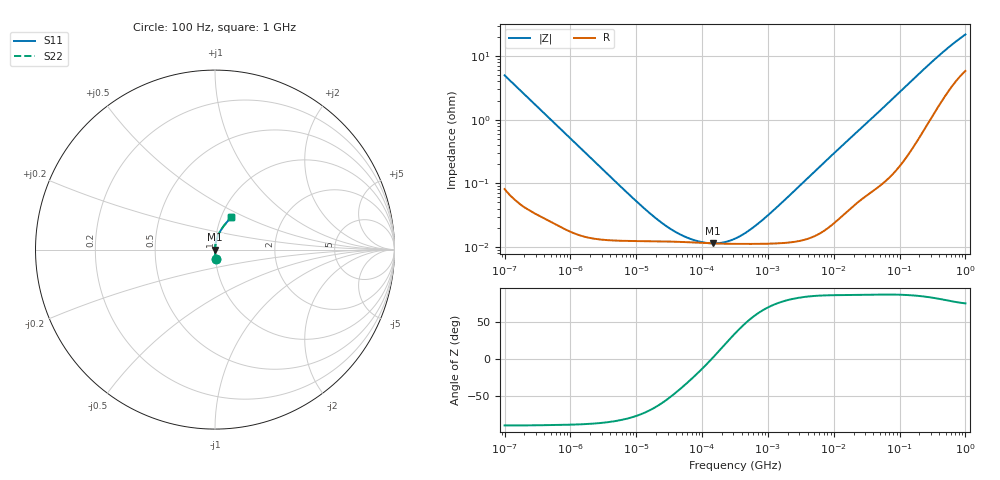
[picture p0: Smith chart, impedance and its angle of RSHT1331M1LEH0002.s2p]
! RSHT1331M1LEH0002  S-PARAMETER MODEL  (General Type)
! Model Generated by ELNA Corporation (http://www.ty-top.com)
! Version 1.0
! ELNA Control No. 201215
! Copyright (c) 2020 ELNA CO.,LTD. All Rights Reserved.
! Products Name : CONDUCTIVE POLYMER HYBRID ALUMINUM ELECTROLYTIC CAPACITORS
! Characteristics :
!  Capacitance  :  330uF  ,  Rated voltage  :  10V
!  Operating Temp. Range  :  -55 to +105 degC  ,  Endurance  :  5000hr at 105 degC
!  Dimension D  :  8mm  ,  Dimension L  :  10mm
! Frequency Range : 100Hz - 1GHz
! External Node Assignments :
!  1  o---| |---o  2
# MHz S RI R 50
!Freq[MHz].  S11 Real  S11 Imag  S21 Real  S21 Imag  S12 Real  S12 Imag  S22 Real  S22 Imag
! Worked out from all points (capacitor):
!   401 points, 100 Hz to 1 GHz, reference 50 ohm
!   read as one part in series: C = 318 uF near 108 Hz
!   lowest |Z| = 11.3 mohm at 147.1 kHz (marker M1)
!   series resonance near 139.7 kHz, so ESL is about 4.1 nH
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0.0001  0.0033 -0.0498  0.9967 0.0498  0.9967 0.0498  0.0033 -0.0498
0.000113  0.00266 -0.0442  0.9973 0.0442  0.9973 0.0442  0.00266 -0.0442
0.000285  0.000646 -0.0176  0.9994 0.0176  0.9994 0.0176  0.000646 -0.0176
0.001488  0.00016 -0.00342  0.9998 0.00342  0.9998 0.00342  0.00016 -0.00342
0.00912  0.000124 -0.000558  0.9999 0.000558  0.9999 0.000558  0.000124 -0.000558
0.014791  0.000123 -0.000343  0.9999 0.000343  0.9999 0.000343  0.000123 -0.000343
0.022131  0.000122 -0.000227  0.9999 0.000227  0.9999 0.000227  0.000122 -0.000227
0.035892  0.000121 -0.000136  0.9999 0.000136  0.9999 0.000136  0.000121 -0.000136
0.05821  0.000119 -7.61e-05  0.9999 7.61e-05  0.9999 7.61e-05  0.000119 -7.61e-05
0.094406  0.000116 -3.19e-05  0.9999 3.19e-05  0.9999 3.19e-05  0.000116 -3.19e-05
0.147062  0.000113 4.17e-06  0.9999 -4.17e-06  0.9999 -4.17e-06  0.000113 4.17e-06
0.220039  0.000112 3.87e-05  0.9999 -3.87e-05  0.9999 -3.87e-05  0.000112 3.87e-05
0.316228  0.000111 7.56e-05  0.9999 -7.56e-05  0.9999 -7.56e-05  0.000111 7.56e-05
0.492606  0.000111 0.000135  0.9999 -0.000135  0.9999 -0.000135  0.000111 0.000135
0.798914  0.000112 0.000231  0.9999 -0.000231  0.9999 -0.000231  0.000112 0.000231
1.522299  0.000114 0.000451  0.9999 -0.000451  0.9999 -0.000451  0.000114 0.000451
4.704354  0.000144 0.0014  0.9999 -0.0014  0.9999 -0.0014  0.000144 0.0014
69.9842  0.00159 0.019  0.9984 -0.019  0.9984 -0.019  0.00159 0.019
176.8072  0.00647 0.0468  0.9935 -0.0468  0.9935 -0.0468  0.00647 0.0468
380.1894  0.0243 0.0934  0.9757 -0.0934  0.9757 -0.0934  0.0243 0.0934
668.3439  0.0569 0.1422  0.9431 -0.1422  0.9431 -0.1422  0.0569 0.1422
1000  0.0916 0.1815  0.9084 -0.1815  0.9084 -0.1815  0.0916 0.1815
